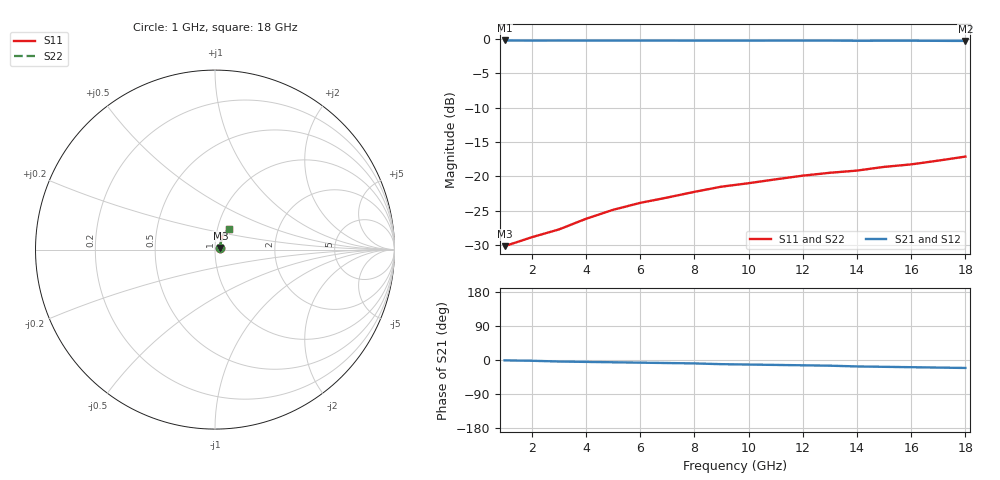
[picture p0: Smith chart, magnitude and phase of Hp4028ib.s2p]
!HPND-4028 beam lead PIN diode
!Series configuration S-parameters If=5 mA.  Last updated 10/3/97
# mhz s ma r 50
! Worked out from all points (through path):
!   18 points, 1 GHz to 18 GHz, reference 50 ohm
!   highest |S21| = -0.24 dB at 1 GHz (marker M1); lowest = -0.3 dB at 18 GHz (marker M2)
!   group delay of S21, straight-line fit = 3.29 ps
!   lowest |S11| = -30.2 dB at 1 GHz (marker M3), VSWR 1.06, Z = 53 + j0.962 ohm
!   |S11| at or under -10 dB: start of sweep to end of sweep
!   |S22| runs from -30.2 to -17.1 dB; largest |S21 - S12| = 0
1000  0.031 17.0  0.973 -1.0  0.973 -1.0  0.031 17.0
2000  0.036 33.0  0.971 -2.0  0.971 -2.0  0.036 33.0
3000  0.041 43.0  0.972 -4.0  0.972 -4.0  0.041 43.0
4000  0.049 49.0  0.971 -5.0  0.971 -5.0  0.049 49.0
5000  0.057 54.0  0.971 -6.0  0.971 -6.0  0.057 54.0
6000  0.064 57.0  0.971 -7.0  0.971 -7.0  0.064 57.0
7000  0.07 60.0  0.971 -8.0  0.971 -8.0  0.07 60.0
8000  0.077 60.0  0.97 -9.0  0.97 -9.0  0.077 60.0
9000  0.084 61.0  0.97 -11.0  0.97 -11.0  0.084 61.0
10000  0.089 61.0  0.97 -12.0  0.97 -12.0  0.089 61.0
11000  0.095 61.0  0.971 -13.0  0.971 -13.0  0.095 61.0
12000  0.101 60.0  0.971 -14.0  0.971 -14.0  0.101 60.0
13000  0.106 59.0  0.971 -15.0  0.971 -15.0  0.106 59.0
14000  0.11 59.0  0.968 -17.0  0.968 -17.0  0.11 59.0
15000  0.117 58.0  0.969 -18.0  0.969 -18.0  0.117 58.0
16000  0.122 57.0  0.969 -19.0  0.969 -19.0  0.122 57.0
17000  0.13 56.0  0.967 -20.0  0.967 -20.0  0.13 56.0
18000  0.139 55.0  0.965 -21.0  0.965 -21.0  0.139 55.0
